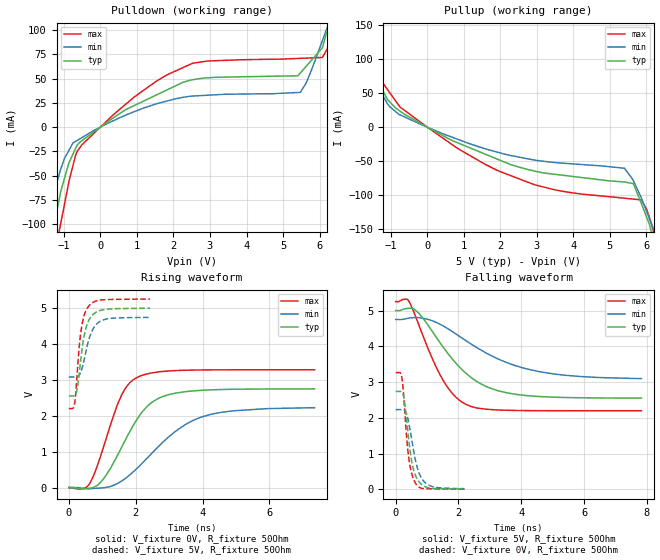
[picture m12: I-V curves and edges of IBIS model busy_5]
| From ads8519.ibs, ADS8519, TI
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|   busy_5 Model
[Model]   busy_5
Model_type   Output
Polarity   Non-Inverting
Vmeas = 2.5
Vref = 2.5
Cref = 5pF
Rref = 50
|   typ   min   max
|   (nom PVT)   (Fast PVT)   (slow PVT)
| C_comp by Frequency method (F=29Mhz)
|Average
|C_comp   5.311e-12   4.488e-12   6.381e-12
|ON state : BUFFER OUTPUT TURNED HIGH
|C_comp   5.311e-12   4.488e-12   6.381e-12
|OFF state: BUFFER OUTPUT TURNED LOW
|C_comp   5.556e-12   4.916e-12   6.389e-12
| C_comp by LC Tank method (L=1nH)
| Resonant frequency (Hz)  2.98e9   3.24e9   2.76e9
C_comp   2.855e-12   2.408e-12   3.329e-12
| Where nom  PVT is Nominal Process,  5V,  32C
|   Fast PVT is Strong Process,   5.25V,  -40C
|   Slow PVT is Weak Process,   4.75V,  92C
[Voltage Range]   5   4.75   5.25
|Ambient Temperature   25   85   -40
|Junction Temperature
[Temperature Range]   32   92   -40
[Pullup Reference]   5   4.75   5.25
[Pulldown Reference]   0   0   0
[Power Clamp Reference]   5   4.75   5.25
[GND Clamp Reference]   0   0   0
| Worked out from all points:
|   slope of the pulldown table from 0 to 0.75 V, typ, clamps not added: 39.4 ohm
|   slope of the pullup table from 0 to 0.75 V, typ, clamps not added: 35.3 ohm
|   falling waveform, V_fixture 5V, R_fixture 50Ohm: 20-80 % time 1.45ns typ, 2.15ns min, 970ps max; typ from 5 V to 2.55 V
|   rising waveform, V_fixture 0V, R_fixture 50Ohm: 20-80 % time 1.03ns typ, 1.6ns min, 735ps max; typ from 0 V to 2.75 V
|   rising waveform, V_fixture 5V, R_fixture 50Ohm: 20-80 % time 239ps typ, 296ps min, 195ps max; typ from 2.55 V to 4.99 V
|   falling waveform, V_fixture 0V, R_fixture 50Ohm: 20-80 % time 249ps typ, 309ps min, 200ps max; typ from 2.74 V to 0.013 V
[Pulldown]
|   Voltage   I(typ)   I(min)   I(max)
-5V       -973.2mA   -710.1mA   -1.337A
-1.833V   -226.6mA   -149.4mA   -323.7mA
-1.306V   -108.1mA   -71.2mA    -155mA
-1.129V   -74.51mA   -48.77mA   -107.4mA
-677.3mV  -21.75mA   -14.64mA   -28.84mA
-509.2mV  -14.03mA   -10.87mA   -18.29mA
2.525V    48.75mA    31.98mA    65.74mA
5.472V    55.68mA    35.76mA    70.77mA
6.075V    81.51mA    88.76mA    71.7mA
6.237V    103mA      105.3mA    82.31mA
6.525V    140.9mA    134.7mA    130.7mA
10V       373.1mA    321.6mA    437.7mA
[Pullup]
|   Voltage   I(typ)   I(min)   I(max)
-5V       293.4mA    260.7mA    340.9mA
-2.562V   185.3mA    160.3mA    219.1mA
-1.953V   136.1mA    116mA      162.7mA
-1.307V   62.64mA    54.64mA    71.85mA
-865mV    28.18mA    22.79mA    38.58mA
924mV     -25.07mA   -19.7mA    -34.31mA
2.94V     -64.75mA   -48.53mA   -84.86mA
5.396V    -80.72mA   -60.49mA   -104.6mA
5.65V     -83.77mA   -79.79mA   -106mA
5.87V     -113.8mA   -105.5mA   -107.6mA
6.184V    -164.5mA   -148.8mA   -151.4mA
10V       -1.065A    -823.3mA   -1.37A
[Ramp]
R_load = 50
|   typ   min   max
dV/dt_r   1.64871/1.02701e-09   1.33984/1.6098e-09   1.96698/7.3468e-10
dV/dt_f   1.46981/1.44895e-09   1.00069/2.18427e-09   1.83103/9.70004e-10
[Falling Waveform]
V_fixture = 5V
V_fixture_min = 4.75V
V_fixture_max = 5.25V
R_fixture = 50Ohm
|   Time   V(typ)   V(min)   V(max)
0s        5V         4.75V      5.25V
405ps     5.063V     4.788V     5.282V
765ps     4.898V     4.8V       4.535V
1.17ns    4.413V     4.715V     3.65V
1.5ns     3.994V     4.577V     3.067V
1.905ns   3.542V     4.354V     2.589V
2.25ns    3.238V     4.152V     2.373V
3.165ns   2.785V     3.687V     2.225V
4.47ns    2.602V     3.311V     2.201V
7.83ns    2.552V     3.097V     2.198V
[Rising Waveform]
V_fixture = 0V
V_fixture_min = 0V
V_fixture_max = 0V
R_fixture = 50Ohm
|   Time   V(typ)   V(min)   V(max)
0s        1.662nV    1.976nV    1.465nV
435ps     -37.6mV    -21.2mV    -25.66mV
630ps     -17.7mV    -33.07mV   124.9mV
1.05ns    257.5mV    -4.833mV   1.167V
1.575ns   1.115V     179.6mV    2.565V
1.815ns   1.543V     346.8mV    2.907V
2.115ns   2.004V     604.7mV    3.097V
2.805ns   2.532V     1.255V     3.232V
3.975ns   2.707V     1.966V     3.274V
7.35ns    2.747V     2.223V     3.278V
[Rising Waveform]
V_fixture = 5V
V_fixture_min = 4.75V
V_fixture_max = 5.25V
R_fixture = 50Ohm
|   Time   V(typ)   V(min)   V(max)
0s        2.55V      3.078V     2.198V
165ps     2.556V     3.078V     2.299V
210ps     2.609V     3.077V     2.661V
255ps     2.777V     3.085V     3.236V
360ps     3.579V     3.217V     4.326V
450ps     4.181V     3.518V     4.763V
570ps     4.598V     4.022V     5.019V
750ps     4.839V     4.455V     5.169V
1.005ns   4.944V     4.656V     5.226V
2.43ns    4.991V     4.737V     5.246V
[Falling Waveform]
V_fixture = 0V
V_fixture_min = 0V
V_fixture_max = 0V
R_fixture = 50Ohm
|   Time   V(typ)   V(min)   V(max)
0s        2.738V     2.23V      3.265V
195ps     2.723V     2.23V      3.131V
285ps     2.429V     2.206V     2.242V
345ps     1.981V     2.115V     1.498V
405ps     1.476V     1.915V     953.1mV
510ps     785.5mV    1.391V     442mV
630ps     387mV      812.6mV    175.9mV
795ps     159.7mV    358.5mV    38.57mV
1.02ns    49.09mV    134.5mV    15.52mV
2.19ns    12.72mV    20.61mV    4.928mV
